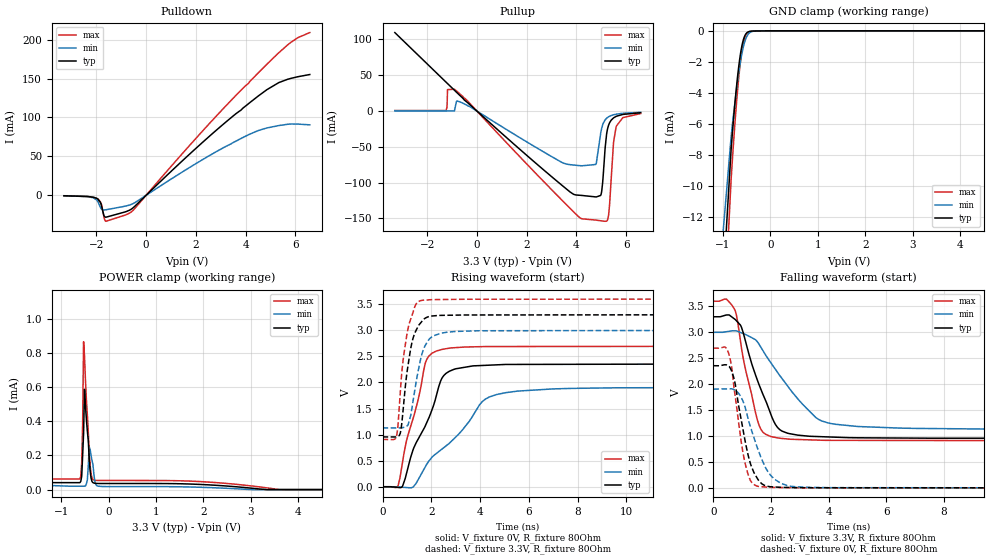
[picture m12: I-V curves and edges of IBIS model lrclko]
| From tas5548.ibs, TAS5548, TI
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|   lrcko Model
[Model]   lrclko
Model_type   I/O
Polarity   Non-Inverting
Enable   Active-Low
Vinl = 0.8
Vinh = 2.0
Vmeas = 1.65
Vref = 0
Cref = 1pF
Rref = 1000000
|   typ   min   max
C_comp   1.035pF   0.913pF   1.101pF
[Voltage Range]   3.3   3   3.6
[Temperature Range]   27   125   0
[Pullup Reference]   3.3   3   3.6
[Pulldown Reference]   -0   -0   -0
[Power Clamp Reference]   3.3   3   3.6
[GND Clamp Reference]   -0   -0   -0
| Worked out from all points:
|   slope of the pulldown table from 0 to 0.495 V, typ, clamps not added: 32.5 ohm
|   slope of the pullup table from 0 to 0.495 V, typ, clamps not added: 31.9 ohm
|   GND clamp passes 1 mA (typ) near -0.60 V on its own axis
|   POWER clamp passes 1 mA (typ) near -3.27 V on its own axis
|   falling waveform, V_fixture 3.3V, R_fixture 80Ohm: 20-80 % time 877ps typ, 1.55ns min, 583ps max; typ from 3.3 V to 0.956 V
|   rising waveform, V_fixture 0V, R_fixture 80Ohm: 20-80 % time 1.18ns typ, 2.16ns min, 816ps max; typ from 0 V to 2.35 V
|   rising waveform, V_fixture 3.3V, R_fixture 80Ohm: 20-80 % time 407ps typ, 468ps min, 384ps max; typ from 0.956 V to 3.3 V
|   falling waveform, V_fixture 0V, R_fixture 80Ohm: 20-80 % time 492ps typ, 703ps min, 405ps max; typ from 2.35 V to 0 V
[Pulldown]
|   Voltage   I(typ)   I(min)   I(max)
-3.3V     -560uA     -542.7uA   -599.6uA
-2.33V    -1.558mA   -1.766mA   -1.617mA
-1.954V   -4.503mA   -7.424mA   -4.367mA
-1.815V   -10.87mA   -16.78mA   -9.794mA
-1.696V   -25.85mA   -18.83mA   -27.49mA
-1.617V   -28.14mA   -18.58mA   -33.37mA
-627mV    -18.41mA   -12.03mA   -22.03mA
2.284V    68.44mA    46.11mA    83.07mA
4.184V    119.5mA    78.82mA    146.8mA
5.333V    144.8mA    89.61mA    183.1mA
6.105V    152.4mA    91.48mA    202.6mA
6.58V     155.2mA    90.54mA    209.1mA
[GND Clamp]
|   Voltage   I(typ)   I(min)   I(max)
-3.3V     -1.514A    -1.357A    -1.56A
-1.617V   -48.03mA   -35.56mA   -57.75mA
-825mV    -7.62mA    -6.822mA   -9.54mA
-726mV    -4.041mA   -4.122mA   -5.196mA
-666.6mV  -2.339mA   -2.741mA   -3.077mA
-627mV    -1.458mA   -1.957mA   -1.947mA
-587.4mV  -809.7uA   -1.304mA   -1.094mA
-547.8mV  -395.5uA   -799.4uA   -533.3uA
-468.6mV  -73.01uA   -226.6uA   -92.75uA
-389.4mV  -18.6uA    -49.79uA   -22.84uA
-211.2mV  -6.759uA   -4.197uA   -8.797uA
6.58V     0A         0A         0A
[Pullup]
|   Voltage   I(typ)   I(min)   I(max)
-3.3V     109.6mA    165.8uA    758.3uA
-1.241V   40.37mA    144.4uA    708.1uA
-1.181V   38.36mA    144.3uA    29.94mA
-904.2mV  29.06mA    146.5uA    30.43mA
3.887V    -116.3mA   -75.41mA   -140.8mA
4.778V    -119.9mA   -74.6mA    -152.3mA
4.976V    -117.8mA   -30.69mA   -153.3mA
5.155V    -50.95mA   -12.31mA   -154mA
5.293V    -19.68mA   -7.98mA    -145.2mA
5.491V    -9.555mA   -5.225mA   -43.84mA
5.61V     -7.23mA    -4.311mA   -20.75mA
6.58V     -2.367mA   -1.746mA   -3.502mA
[POWER Clamp]
|   Voltage   I(typ)   I(min)   I(max)
-3.3V     1.08mA     9.274mA    1.113mA
-2.864V   508.9uA    1.139mA    537.9uA
-2.686V   344.5uA    525uA      331.2uA
-2.31V    87.56uA    249.8uA    78.69uA
-1.657V   40.96uA    28.33uA    62.57uA
-607.2mV  40.65uA    19.96uA    62.06uA
-567.6mV  76.96uA    19.95uA    156uA
-528mV    327.4uA    19.95uA    864.7uA
-508.2mV  586.9uA    19.95uA    779.6uA
-389.4mV  107.6uA    234.8uA    140.8uA
-310.2mV  38.38uA    87.41uA    56.14uA
6.58V     0A         0A         0A
[Ramp]
R_load = 80
|   typ   min   max
dV/dt_r   1.41322/1.18466e-09   1.14234/2.15903e-09   1.61634/8.17132e-10
dV/dt_f   1.40597/8.76866e-10   1.1223/1.54928e-09   1.61456/5.83119e-10
[Falling Waveform]
V_fixture = 3.3V
V_fixture_min = 3V
V_fixture_max = 3.6V
R_fixture = 80Ohm
C_fixture = 0F
|   Time   V(typ)   V(min)   V(max)
0s        3.299V     2.999V     3.599V
453.9ps   3.333V     3.011V     3.639V
760.4ps   3.245V     3.028V     3.411V
973.4ps   3.099V     2.989V     2.703V
1.536ns   2.063V     2.81V      1.292V
1.969ns   1.457V     2.433V     995mV
2.38ns    1.095V     2.11V      952.7mV
3.553ns   990.5mV    1.357V     922mV
4.093ns   979.9mV    1.239V     915.9mV
15ns      955.9mV    1.129V     908mV
[Rising Waveform]
V_fixture = 0V
V_fixture_min = 0V
V_fixture_max = 0V
R_fixture = 80Ohm
C_fixture = 0F
|   Time   V(typ)   V(min)   V(max)
0s        586.3nV    22.15uV    -25.21nV
638.3ps   -13.44mV   -3.641mV   20.33mV
825.8ps   15.69mV    -10.1mV    487.1mV
1.235ns   683.4mV    -10.89mV   1.281V
1.741ns   1.154V     371.2mV    2.348V
2.206ns   1.745V     637.4mV    2.603V
2.744ns   2.216V     836.4mV    2.658V
4.093ns   2.326V     1.635V     2.688V
4.743ns   2.34V      1.775V     2.69V
15ns      2.355V     1.904V     2.694V
[Rising Waveform]
V_fixture = 3.3V
V_fixture_min = 3V
V_fixture_max = 3.6V
R_fixture = 80Ohm
C_fixture = 0F
|   Time   V(typ)   V(min)   V(max)
0s        955.9mV    1.129V     908mV
570.7ps   957.7mV    1.129V     955.2mV
729.4ps   1.029V     1.129V     1.821V
850.3ps   1.503V     1.137V     2.452V
1.03ns    2.28V      1.179V     2.998V
1.25ns    2.846V     1.638V     3.345V
1.536ns   3.128V     2.393V     3.566V
1.939ns   3.269V     2.844V     3.587V
2.627ns   3.289V     2.963V     3.593V
15ns      3.299V     2.999V     3.599V
[Falling Waveform]
|Gnd
V_fixture = 0V
V_fixture_min = 0V
V_fixture_max = 0V
R_fixture = 80Ohm
C_fixture = 0F
|   Time   V(typ)   V(min)   V(max)
0s        2.355V     1.904V     2.694V
520.6ps   2.352V     1.91V      2.611V
620.8ps   2.269V     1.911V     2.373V
729.4ps   2.078V     1.891V     1.879V
1.079ns   971.7mV    1.592V     529.8mV
1.279ns   481.3mV    1.189V     150.4mV
1.499ns   207mV      816.1mV    36.41mV
1.986ns   21.59mV    241.3mV    9.167mV
2.722ns   6.274mV    27.61mV    3.611mV
15ns      584nV      21.97uV    -63.15nV
